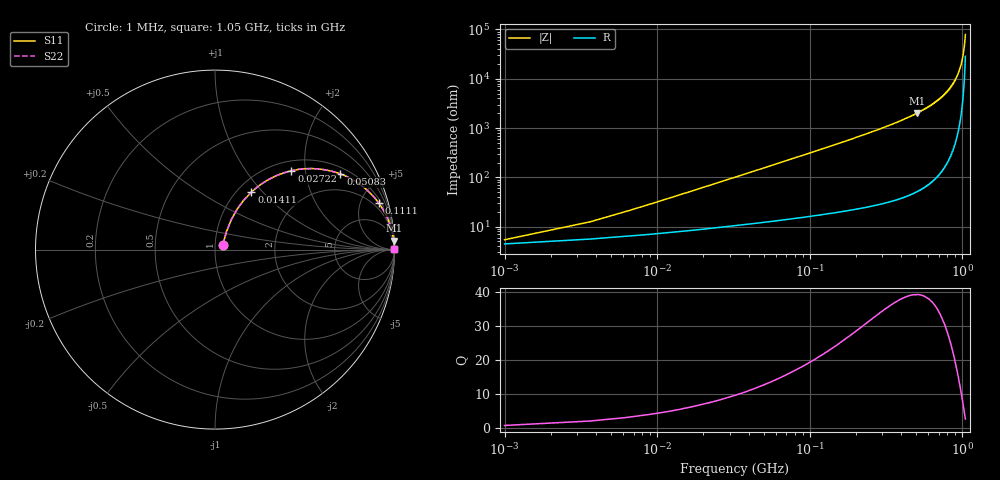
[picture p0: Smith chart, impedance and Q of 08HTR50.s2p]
! Coilcraft 0805HT-R50 Chip Inductor
! 6 August 2004
# MHZ S MA R 50
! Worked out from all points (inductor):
!   401 points, 1 MHz to 1.05 GHz, reference 50 ohm
!   read as one part in series: L = 491 nH near 6.245 MHz
!   highest Q = 39.3 at 507.1 MHz (marker M1), where L = 639 nH
!   S11 on the Smith chart (normalised r, x): 1 MHz: 1.09, +0.06; 14.11 MHz: 1.16, +0.87; 27.23 MHz: 1.20, +1.68; 50.83 MHz: 1.25, +3.14; 111.1 MHz: 1.33, +6.94; 1.05 GHz: open
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1  0.052 32.9  0.957 -1.7  0.957 -1.7  0.052 32.9
3.623  0.118 57.3  0.942 -6.0  0.942 -6.0  0.118 57.3
8.867  0.256 61.3  0.906 -14.3  0.906 -14.3  0.256 61.3
14.112  0.38 57.7  0.859 -22.0  0.859 -22.0  0.38 57.7
19.357  0.487 52.9  0.806 -28.8  0.806 -28.8  0.487 52.9
27.225  0.612 45.9  0.723 -37.4  0.723 -37.4  0.612 45.9
37.715  0.727 38.2  0.621 -46.4  0.621 -46.4  0.727 38.2
50.828  0.816 31.1  0.518 -54.5  0.518 -54.5  0.816 31.1
77.053  0.904 22.1  0.377 -64.4  0.377 -64.4  0.904 22.1
111.145  0.949 15.8  0.273 -71.4  0.273 -71.4  0.949 15.8
176.708  0.978 10.0  0.174 -77.8  0.174 -77.8  0.978 10.0
260.628  0.99 6.6  0.116 -81.6  0.116 -81.6  0.99 6.6
352.415  0.994 4.7  0.082 -83.8  0.082 -83.8  0.994 4.7
507.143  0.998 2.8  0.049 -85.7  0.049 -85.7  0.998 2.8
525.5  0.998 2.7  0.047 -85.9  0.047 -85.9  0.998 2.7
701.207  0.999 1.5  0.026 -86.8  0.026 -86.8  0.999 1.5
811.352  0.999 1.0  0.017 -86.9  0.017 -86.9  0.999 1.0
876.915  0.999 0.7  0.012 -86.7  0.012 -86.7  0.999 0.7
942.477  0.999 0.4  0.007751 -85.8  0.007751 -85.8  0.999 0.4
989.682  1 0.3  0.004786 -83.9  0.004786 -83.9  1 0.3
1023.775  1 0.2  0.002748 -80.1  0.002748 -80.1  1 0.2
1050  1 0.1  0.001262 -68.9  0.001262 -68.9  1 0.1
